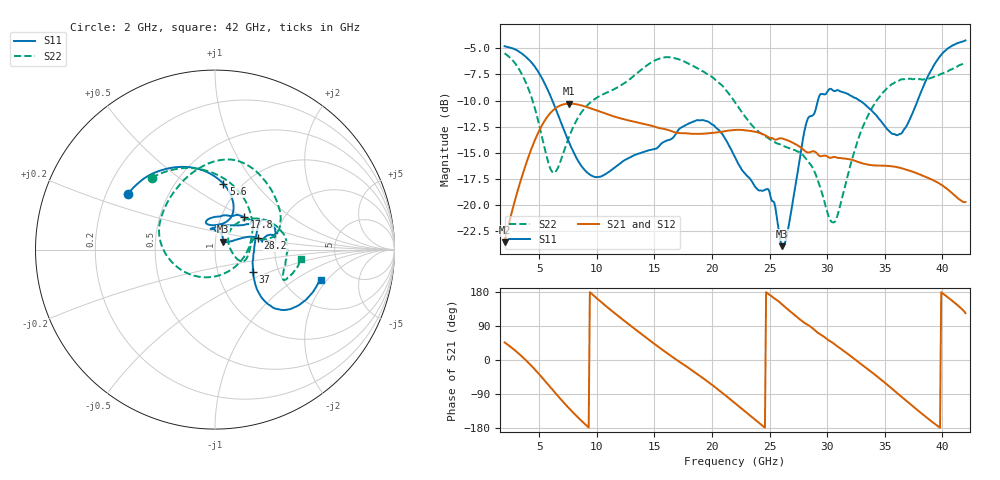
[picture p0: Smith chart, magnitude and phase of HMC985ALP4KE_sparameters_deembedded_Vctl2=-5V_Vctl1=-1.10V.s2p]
!s2p File: Measurements: S11, S21, S12, S22
# GHz S dB R 50.0
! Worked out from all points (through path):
!   401 points, 2 GHz to 42 GHz, reference 50 ohm
!   highest |S21| = -10.29 dB at 7.6 GHz (marker M1); lowest = -23.6 dB at 2 GHz (marker M2)
!   lowest |S11| = -24.0 dB at 26.1 GHz (marker M3), VSWR 1.14, Z = 54.6 + j4.82 ohm
!   |S11| at or under -10 dB: 6.148 GHz to 29.2 GHz (23.05 GHz wide, 130 % of centre); 32.8 GHz to 37.85 GHz (5.055 GHz wide, 14.3 % of centre)
!   |S22| runs from -21.7 to -5.5 dB; largest |S21 - S12| = 0.00035
!   S11 on the Smith chart (normalised r, x): 2 GHz: 0.29, +0.27; 5.6 GHz: 0.83, +0.70; 17.8 GHz: 1.28, +0.49; 28.2 GHz: 1.61, +0.22; 37 GHz: 1.47, -0.39; 42 GHz: 3.17, -1.72
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2  -4.79 147.8  -23.61 46.5  -23.62 46.5  -5.46 131.4
3.6  -5.58 121.2  -16.95 6.6  -16.95 6.6  -7.70 86.8
4.7  -6.88 100.3  -13.61 -27.4  -13.62 -27.4  -11.03 45.0
5.6  -8.64 82.8  -11.73 -58.6  -11.73 -58.6  -15.15 -7.0
6.4  -10.70 70.3  -10.75 -87.0  -10.76 -87.0  -16.86 -73.8
7.6  -14.02 63.7  -10.29 -127.6  -10.30 -127.6  -13.46 -145.0
8.7  -16.32 72.8  -10.47 -161.2  -10.48 -161.2  -11.08 -176.4
12  -16.05 108.5  -11.69 112.7  -11.69 112.8  -8.61 136.5
15.4  -14.38 79.2  -12.63 33.7  -12.64 33.7  -5.99 85.5
17.8  -12.31 48.2  -13.14 -17.3  -13.15 -17.3  -6.38 57.0
20  -12.29 36.3  -13.10 -65.5  -13.11 -65.5  -7.73 27.0
22  -15.42 53.0  -12.82 -114.0  -12.82 -114.0  -10.16 11.6
24.9  -18.52 96.6  -13.51 174.2  -13.52 174.3  -13.62 11.2
26.1  -23.96 43.9  -13.64 146.3  -13.64 146.3  -14.29 -1.8
28.2  -12.12 15.0  -14.94 94.8  -14.94 94.8  -15.62 -23.4
28.7  -11.45 9.7  -14.87 84.5  -14.88 84.6  -16.35 -24.1
30.6  -9.09 16.3  -15.41 42.6  -15.41 42.7  -21.67 20.8
33  -10.12 31.5  -16.00 -12.1  -16.01 -12.0  -12.77 45.9
35.4  -12.94 9.3  -16.28 -69.9  -16.28 -69.8  -8.64 19.9
37  -12.20 -30.6  -16.67 -110.8  -16.67 -110.8  -7.91 1.4
39.6  -6.07 -42.4  -17.86 -174.4  -17.87 -174.4  -7.61 -23.7
42  -4.24 -16.0  -19.73 123.7  -19.74 123.8  -6.37 -6.1
